// TwinCAT 3 PLC project OOP3_Generator
// ProgramVersion: 3.1.4020.2
// libraries:
//   Tc2_Standard, * (Beckhoff Automation GmbH)
//   Tc2_System, * (Beckhoff Automation GmbH)
//   Tc3_Module, * (Beckhoff Automation GmbH)
// project tree:
//   / PlcTask.TcTTO
//   POUs/ FB_Generator.TcPOU, FB_GeneratorEX.TcPOU, I_Generator.TcIO, MAIN.TcPOU

CONFIGURATION OOP3_Generator
    RESOURCE PLC ON TwinCAT3
        TASK PlcTask(INTERVAL := T#10ms, PRIORITY := 20);
        PROGRAM MAIN WITH PlcTask : MAIN;
    END_RESOURCE
END_CONFIGURATION

// ---- POUs/I_Generator.TcIO
INTERFACE I_Generator

METHOD M_Flash : BOOL
VAR_INPUT
END_VAR
END_METHOD

PROPERTY P_Cycletime : TIME
GET
END_GET
SET
END_SET
END_PROPERTY

PROPERTY P_Vendor : String
GET
END_GET
END_PROPERTY

END_INTERFACE

// ---- POUs/MAIN.TcPOU
PROGRAM MAIN
VAR
	change: BOOL:=TRUE;
	IGenerator:I_Generator;
	FBGenerator1: FB_Generator;
	FBGenerator2: FB_GeneratorEX;
	input: BOOL;
	tCycletime: TIME:=t#3S;
	sVendor: STRING;
	
END_VAR

IF change THEN
	IGenerator:=FBGenerator1;
ELSE
	IGenerator:=FBGenerator2;
END_IF
				
input := IGenerator.M_Flash();
sVendor:=IGenerator.P_Vendor;
IGenerator.P_Cycletime:=tCycletime;

END_PROGRAM

// ---- POUs/FB_Generator.TcPOU
FUNCTION_BLOCK FB_Generator IMPLEMENTS I_Generator
VAR_INPUT
END_VAR
VAR_OUTPUT
END_VAR
VAR
	tCycletime: TIME;
	fbTon1: TON;
	bFlashVar: BOOL;
END_VAR

{warning 'add method implementation'}
METHOD M_Flash : BOOL
fbTon1(IN:=NOT fbTon1.Q , 
	PT:=tCycletime , 
	Q=> , 
	ET=> );

IF fbTon1.Q THEN
	bFlashVar := NOT bFlashVar;
END_IF

M_Flash := bFlashVar;
END_METHOD

{warning 'add property implementation'}
PROPERTY P_Cycletime : TIME
GET
P_Cycletime:=tCycletime;
END_GET
SET
IF P_Cycletime < T#50MS THEN
	tCycletime := T#50MS;
ELSIF P_Cycletime > T#5S THEN
	tCycletime := T#5S;
ELSE
	tCycletime := P_Cycletime;
END_IF
END_SET
END_PROPERTY

{warning 'add property implementation'}
PROPERTY P_Vendor : STRING
GET
P_Vendor := 'Company X';
END_GET
END_PROPERTY

END_FUNCTION_BLOCK

// ---- POUs/FB_GeneratorEX.TcPOU
FUNCTION_BLOCK FB_GeneratorEX EXTENDS FB_Generator
VAR_INPUT
END_VAR
VAR_OUTPUT
END_VAR
VAR
END_VAR

{warning 'add method implementation'}
METHOD M_Flash : BOOL
fbTon1(IN:=NOT fbTon1.Q , 
		PT:=tCycletime , 
		Q=> , ET=> );

// 33% ON 66% OFF
M_Flash := fbTon1.ET < fbTon1.PT / 3 ;
END_METHOD

PROPERTY P_Vendor : STRING
GET
P_Vendor := CONCAT(STR1:='Company Y based on ' , 
       			 STR2:=SUPER^.P_Vendor );
END_GET
END_PROPERTY

END_FUNCTION_BLOCK
